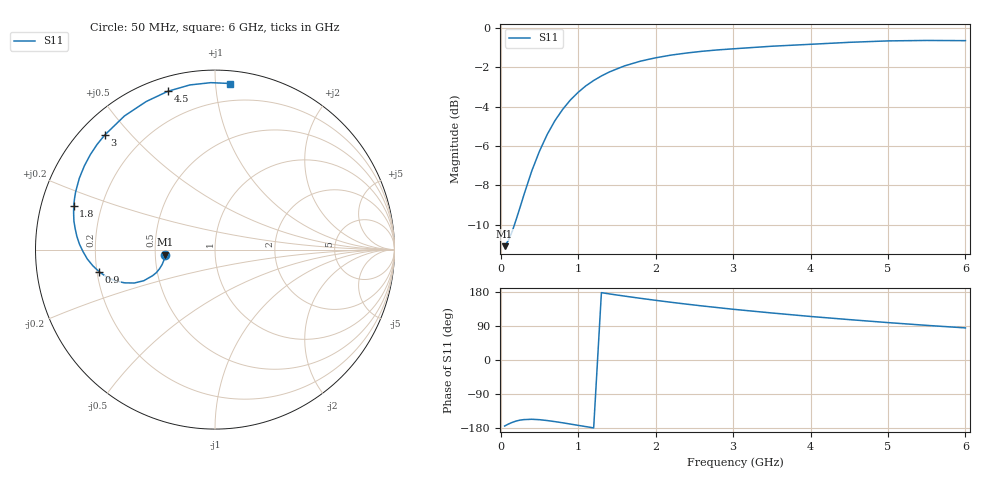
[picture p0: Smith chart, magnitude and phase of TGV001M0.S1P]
! SIEMENS Discrete & RF Semiconductors
! BAT64
! Si Schottky Diode in SOT23
! IF = 1 mA
! S-Parameters:  February  1997
# GHz  S  MA  R  50
!  f  S11
! GHz  MAG  ANG
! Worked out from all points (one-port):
!   34 points, 50 MHz to 6 GHz, reference 50 ohm
!   lowest |S11| = -11.1 dB at 50 MHz (marker M1), VSWR 1.77, Z = 28.2 - j1.73 ohm
!   |S11| at or under -10 dB: start of sweep to 177 MHz
!   S11 on the Smith chart (normalised r, x): 50 MHz: 0.56, -0.03; 900 MHz: 0.21, -0.09; 1.8 GHz: 0.10, +0.15; 3 GHz: 0.07, +0.42; 4.5 GHz: 0.06, +0.74; 6 GHz: 0.08, +1.09
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0.05  0.2789 -174.2
0.1  0.2888 -168.9
0.15  0.3048 -164.5
0.2  0.3263 -161.0
0.3  0.3771 -157.3
0.4  0.4329 -156.4
0.5  0.4864 -157.5
0.6  0.5366 -159.8
0.7  0.5818 -162.6
0.8  0.6215 -165.7
0.9  0.6567 -169.1
1.1  0.7135 -175.8
1.2  0.7359 -179.2
1.4  0.7733 174.5
1.6  0.8019 168.6
1.8  0.8238 162.9
2  0.8405 157.5
2.2  0.854 152.3
2.4  0.8644 147.4
2.6  0.8732 142.7
2.8  0.8803 138.3
3  0.8859 133.9
3.5  0.8995 124.1
4  0.9097 114.9
4.5  0.9203 106.6
5  0.928 98.7
5.5  0.9304 91.4
6  0.9294 84.7
